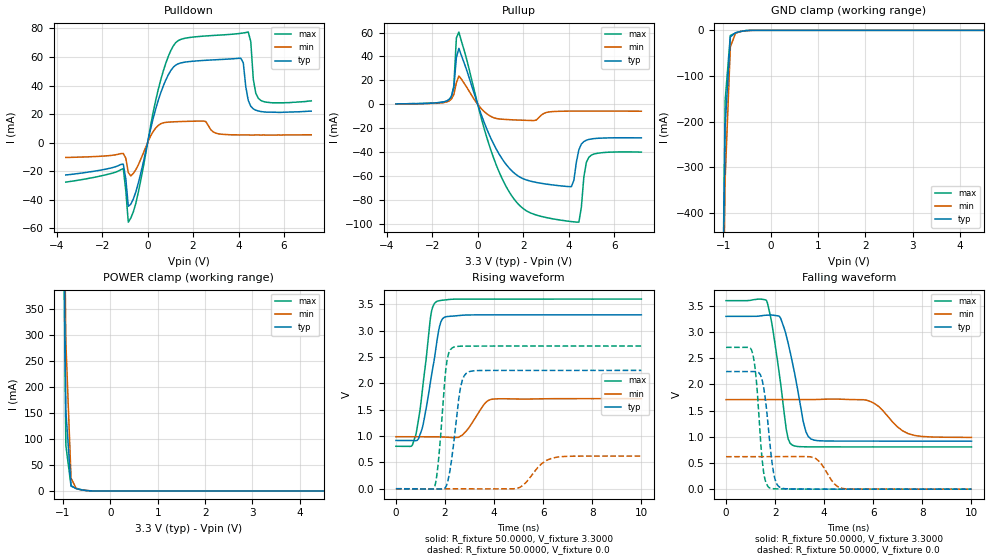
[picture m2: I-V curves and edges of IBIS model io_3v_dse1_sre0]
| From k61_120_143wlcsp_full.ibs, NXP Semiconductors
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[Model]  io_3v_dse1_sre0
|   Model io_3v_dse1_sre0
| Library cells for typ/min/max conditions are connected as defined below:
|  pad - External Pad
|  ipp_do_3v - Core Input
|  ipp_obe_3v - Output Buffer Enable
|  esd_boost - vdd_s_3v
|  esd_trigger - vss_s_3v
|  ipp_ame_3v - vss_s_3v
|  ipp_dse_3v - vdd_s_3v
|  ipp_ina_3v - NC
|  ipp_ina_mux_3v - NC
|  ipp_ind_3v - NC
|  ipp_pue_3v - vss_s_3v
|  ipp_sre_3v - vss_s_3v
|  tie_3v - vdd_s_3v
|  tie_hi - vdd_s_lv
|  vbuf_3v - vdd_s_3v
|  vdd_s_3v - vdd_s_3v
|  vdd_s_lv - vdd_s_lv
|  vss_bulk - vss_s_3v
|  vss_s_3v - vss_s_3v
| All other pins connected to ground
Model_type I/O
Polarity   Non-Inverting
Enable   Active-High
Vinl =   1.1550V
Vinh =   2.3100V
Vmeas =  1.6500V
Cref =   25.0000pF
Rref =   50.0000
Vref =   0.0V
C_comp   1.9040pF   1.7928pF   2.1191pF
[Temperature Range]   25.0000   0.1250k   -40.0000
[Voltage Range]   3.3000V   1.7100V   3.6000V
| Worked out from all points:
|   slope of the pulldown table from 0 to 0.495 V, typ, clamps not added: 16 ohm
|   slope of the pullup table from 0 to 0.495 V, typ, clamps not added: 19.9 ohm
|   GND clamp passes 1 mA (typ) near -0.54 V on its own axis
|   POWER clamp passes 1 mA (typ) near -0.53 V on its own axis
|   rising waveform, R_fixture 50.0000, V_fixture 3.3000: 20-80 % time 498ps typ, 605ps min, 417ps max; typ from 0.916 V to 3.3 V
|   rising waveform, R_fixture 50.0000, V_fixture 0.0: 20-80 % time 352ps typ, 690ps min, 278ps max; typ from 0 V to 2.25 V
|   falling waveform, R_fixture 50.0000, V_fixture 3.3000: 20-80 % time 593ps typ, 894ps min, 483ps max; typ from 3.3 V to 0.917 V
|   falling waveform, R_fixture 50.0000, V_fixture 0.0: 20-80 % time 309ps typ, 516ps min, 259ps max; typ from 2.25 V to 0 V
[Pulldown]
|Voltage   I(typ)   I(min)   I(max)
-3.6V     -22.64mA   -10.39mA   -27.64mA
-1.07V    -15.06mA   -7.583mA   -18.14mA
-850mV    -44.54mA   -20.94mA   -55.71mA
-520mV    -34.63mA   -19mA      -42.63mA
580mV     35mA       13.27mA    44.11mA
1.46V     55.82mA    14.79mA    72.32mA
4.1V      59.16mA    5.4mA      76.58mA
4.43V     29.52mA    5.4mA      77.44mA
4.54V     25.5mA     5.3mA      70.77mA
4.65V     23.68mA    5.3mA      44.58mA
4.87V     22.2mA     5.4mA      31.08mA
7.2V      22.1mA     5.5mA      29.3mA
[Pullup]
|Voltage   I(typ)   I(min)   I(max)
-3.6V     400uA      300uA      500uA
-1.27V    3.86mA     2.75mA     3.76mA
-1.05V    14.15mA    8.34mA     15.69mA
-940mV    39.2mA     18.04mA    55.51mA
-830mV    46.74mA    23.73mA    60.38mA
1.15V     -47.61mA   -12.48mA   -64.99mA
3.13V     -66.86mA   -6.328mA   -94.95mA
4.12V     -68.7mA    -5.62mA    -97.87mA
4.45V     -37.93mA   -5.6mA     -98.38mA
4.78V     -29.93mA   -5.59mA    -48.43mA
5V        -28.86mA   -5.59mA    -42.37mA
7.2V      -27.98mA   -5.71mA    -39.85mA
[GND_clamp]
|Voltage   I(typ)   I(min)   I(max)
-3.6V     -47.78A    -47.06A    -48.3A
-1.07V    -1.101A    -1.183A    -1.105A
-960mV    -210.7mA   -326mA     -154mA
-850mV    -14.47mA   -36.11mA   -11.11mA
-740mV    -5.262mA   -6.034mA   -5.843mA
-520mV    -637uA     -915.4uA   -467.5uA
-300mV    -2.578uA   -18.09uA   -370.9nA
7.2V      0A         0A         0A
[POWER_clamp]
|Voltage   I(typ)   I(min)   I(max)
-3.6V     52.51A     51.88A     52.98A
-1.05V    1.126A     1.265A     1.065A
-940mV    154.2mA    286.1mA    88.03mA
-830mV    9.989mA    24.5mA     9.181mA
-720mV    4.227mA    4.408mA    5.116mA
-390mV    66.57uA    164uA      29.9uA
7.2V      0A         0A         0A
[Ramp]
| variable   typ   min   max
dV/dt_r  1.3476/0.3516n   0.3718/0.6900n   1.6250/0.2777n
dV/dt_f  1.4299/0.5927n   0.4329/0.8942n   1.6762/0.4828n
R_load = 50.0000
[Rising Waveform]
R_fixture= 50.0000
V_fixture= 3.3000
V_fixture_min= 1.7100
V_fixture_max= 3.6000
|time   V(typ)   V(min)   V(max)
0s        916.3mV    987.1mV    805.9mV
621.7ps   914.8mV    987.1mV    805.5mV
792.1ps   911.7mV    987.2mV    993.8mV
1.076ns   1.155V     987.6mV    1.867V
1.43ns    2.093V     987.1mV    3.313V
1.67ns    2.797V     985.6mV    3.556V
1.958ns   3.248V     981.3mV    3.582V
2.71ns    3.293V     1.02V      3.599V
3.873ns   3.3V       1.695V     3.599V
10ns      3.3V       1.71V      3.6V
[Rising Waveform]
R_fixture= 50.0000
V_fixture= 0.0
V_fixture_min= 0.0
V_fixture_max= 0.0
|time   V(typ)   V(min)   V(max)
0s        2.009nV    218.2nV    1.41nV
1.567ns   -4.799mV   12.32uV    24.52mV
1.753ns   -6.838mV   20.88uV    626.9mV
2.042ns   42.34mV    57.6uV     2.304V
2.293ns   631.6mV    87.85uV    2.673V
2.628ns   1.913V     -725uV     2.705V
2.964ns   2.219V     -1.675mV   2.708V
4.978ns   2.246V     13.29mV    2.708V
6.374ns   2.246V     582.4mV    2.708V
10ns      2.246V     619.6mV    2.708V
[Falling Waveform]
R_fixture= 50.0000
V_fixture= 3.3000
V_fixture_min= 1.7100
V_fixture_max= 3.6000
|time   V(typ)   V(min)   V(max)
0s        3.3V       1.71V      3.6V
1.652ns   3.324V     1.71V      3.6V
2.223ns   3.263V     1.71V      2.02V
2.455ns   2.932V     1.71V      1.136V
2.7ns     2.427V     1.71V      840.5mV
3.149ns   1.285V     1.71V      809.3mV
3.466ns   957mV      1.711V     807.9mV
5.717ns   917.2mV    1.701V     806.5mV
7.423ns   916.9mV    1.06V      806.4mV
10ns      916.8mV    988.5mV    806.4mV
[Falling Waveform]
R_fixture= 50.0000
V_fixture= 0.0
V_fixture_min= 0.0
V_fixture_max= 0.0
|time   V(typ)   V(min)   V(max)
0s        2.246V     620mV      2.709V
1.042ns   2.247V     619.9mV    2.655V
1.236ns   2.244V     619.8mV    2.08V
1.465ns   2.096V     619.8mV    590mV
1.751ns   1.039V     619.8mV    30.59mV
1.983ns   211.8mV    619.9mV    7.181mV
2.267ns   19.09mV    620mV      4.72mV
3.66ns    555.8uV    583.9mV    399.4uV
4.787ns   320.3uV    10.23mV    349.5uV
10ns      245.8uV    111.4uV    266.6uV
